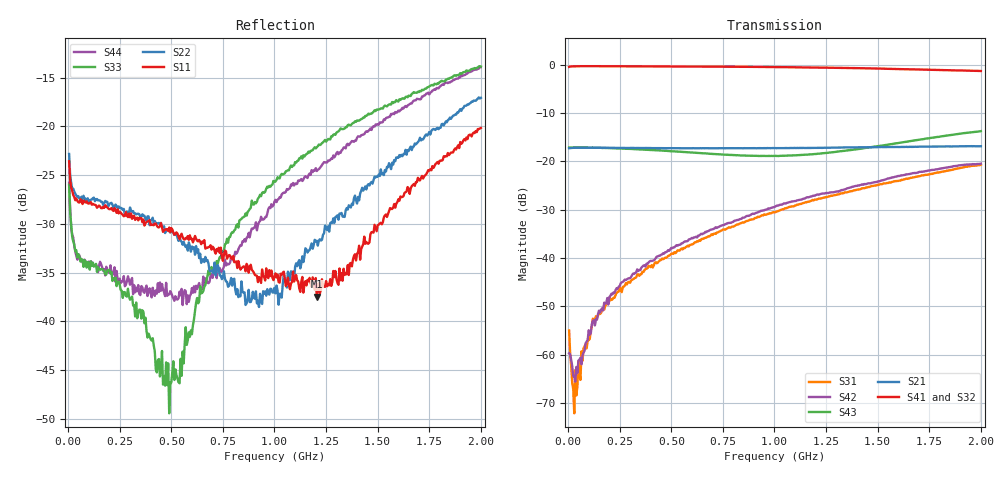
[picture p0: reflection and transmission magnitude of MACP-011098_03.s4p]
!Agilent Technologies,E5071C,MY46110647,A.11.31
!Date: Thu Jul 21 11:38:45 2022
!Data & Calibration Information:
!MACP-011098 solderedd onto PT-0003645 with F connectors, Port1 (pin3) Port2 (pin1) Port3 (pin6) Port4 (pin4)
!Freq	S11:SOLT4(ON)	S12:SOLT4(ON)	S13:SOLT4(ON)	S14:SOLT4(ON)
!	S21:SOLT4(ON)	S22:SOLT4(ON)	S23:SOLT4(ON)	S24:SOLT4(ON)
!	S31:SOLT4(ON)	S32:SOLT4(ON)	S33:SOLT4(ON)	S34:SOLT4(ON)
!	S41:SOLT4(ON)	S42:SOLT4(ON)	S43:SOLT4(ON)	S44:SOLT4(ON)
!PortZ  Port1:75+j0  Port2:75+j0  Port3:75+j0  Port4:75+j0
!Above PortZ is port z conversion or system Z0 setting when saving the data.
!When reading, reference impedance value at option line is always used.
# Hz S MA R 75
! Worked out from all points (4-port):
!   400 points, 5 MHz to 2 GHz, reference 75 ohm
!   strongest paths, dB at 5 MHz, 505 MHz, 1.005 GHz, 1.505 GHz, 2 GHz:
!     S41: -0.5, -0.4, -0.5, -0.8, -1.3
!     S32: -0.4, -0.3, -0.5, -1.0, -1.6
!     S21: -17.3, -17.3, -17.3, -17.1, -16.9
!     S43: -17.1, -17.9, -18.9, -16.8, -13.8
!     S42: -59.7, -38.0, -29.3, -24.1, -20.5
!     S31: -55.0, -39.1, -30.5, -24.8, -20.7
!   lowest |S11| = -37.5 dB at 1.205 GHz (marker M1), VSWR 1.03, Z = 73.3 + j1.08 ohm
!   |S11| at or under -10 dB: start of sweep to end of sweep
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5000000  0.06624 144.5  0.1357 -178.3  0.002065 -83.5  0.9451 2.1
         0.1366 -177.4  0.07219 148.5  0.9489 2.0  0.002796 -93.6
         0.00178 -38.6  0.9516 1.9  0.05013 129.9  0.1378 1.5
         0.9471 2.0  0.001036 -27.1  0.139 1.9  0.05136 133.8
1e7  0.05315 154.4  0.1374 -179.3  0.0005587 -105.5  0.9531 1.1
     0.1372 -179.2  0.05627 154.3  0.954 1.0  0.0007743 -129.7
     0.001033 -47.2  0.9563 1.0  0.03613 141.3  0.1385 0.8
     0.9538 1.1  0.001012 -25.2  0.1386 0.8  0.03813 140.8
3e7  0.04341 165.0  0.1383 178.4  0.0007182 157.8  0.9594 -0.2
     0.1379 178.2  0.04621 165.6  0.9607 -0.2  0.0008863 -172.4
     0.0002482 13.0  0.963 -0.2  0.02476 153.8  0.1389 -0.0
     0.96 -0.2  0.0005987 8.6  0.139 -0.1  0.02447 148.3
1.2e8  0.04004 163.0  0.1388 170.7  0.002531 109.2  0.9619 -3.2
       0.1383 170.8  0.04283 171.4  0.9646 -3.2  0.002374 121.9
       0.002362 92.5  0.9663 -3.2  0.02 159.4  0.1387 -1.7
       0.9629 -3.2  0.002254 83.2  0.1386 -1.8  0.01942 148.8
4.9e8  0.03027 132.7  0.137 142.6  0.01167 88.6  0.9562 -13.8
       0.1366 142.6  0.02892 162.8  0.9612 -14.2  0.01151 96.7
       0.01059 89.4  0.9616 -14.2  0.003373 63.6  0.1275 -5.1
       0.9559 -13.8  0.01187 95.6  0.1277 -5.1  0.01373 85.2
1.205e9  0.01337 146.6  0.1383 91.6  0.04143 57.0  0.9322 -34.5
         0.1379 91.5  0.0259 -136.0  0.9351 -35.6  0.04298 65.6
         0.04043 59.1  0.9294 -35.3  0.07816 -64.6  0.1195 9.3
         0.9312 -34.4  0.04522 67.4  0.1195 9.5  0.05901 -59.8
2e9  0.09825 -166.0  0.1437 28.0  0.09391 0.6  0.8567 -58.6
     0.1433 27.7  0.14 -162.0  0.8382 -61.5  0.09296 11.9
     0.09226 1.6  0.8357 -60.0  0.2028 -120.2  0.2047 6.1
     0.858 -58.4  0.09441 13.5  0.2049 6.2  0.2015 -116.5
